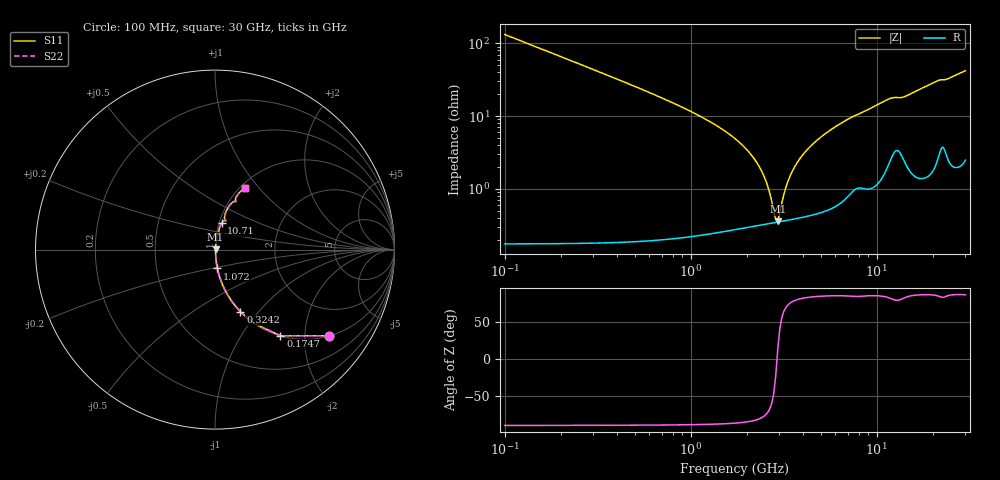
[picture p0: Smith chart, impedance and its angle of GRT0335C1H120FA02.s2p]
!Murata Part Number: GRT0335C1H120FA02
!These Parameters are Measured in Series Mode Connection
!Data Generated on Jun 19, 2026
!  o--ll--o
!Port1  Port2
!  o------o
!Operation Temp=25[degC], DC Bias Voltage=0[V]
!Freq. Start=100[MHz] Stop=30[GHz] 401[Steps]
# Hz S RI R 50
!Freq.(Hz) S11(Real) S11(Imag) S21(Real) S21(Imag) S12(Real) S12(Imag) S22(Real) S22(Imag)
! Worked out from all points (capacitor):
!   401 points, 100 MHz to 30 GHz, reference 50 ohm
!   read as one part in series: C = 12 pF near 249.5 MHz
!   lowest |Z| = 360 mohm at 2.941 GHz (marker M1)
!   series resonance near 2.915 GHz, so ESL is about 250 pH
!   S11 on the Smith chart (normalised r, x): 100 MHz: 1.00, -2.65; 174.8 MHz: 1.00, -1.51; 324.2 MHz: 1.00, -0.81; 1.072 GHz: 1.00, -0.21; 10.71 GHz: 1.03, +0.31; 30 GHz: 1.05, +0.84
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1e8  0.6368 -0.4803  0.3632 0.4803  0.3632 0.4803  0.6368 -0.4803
1.7475e8  0.3641 -0.48  0.6359 0.48  0.6359 0.48  0.3641 -0.48
3.2425e8  0.1413 -0.3461  0.8587 0.3461  0.8587 0.3461  0.1413 -0.3461
5.485e8  0.0531 -0.2201  0.9469 0.2201  0.9469 0.2201  0.0531 -0.2201
1.07175e9  0.0134 -0.1049  0.9866 0.1049  0.9866 0.1049  0.0134 -0.1049
2.193e9  0.00373 -0.0258  0.9963 0.0258  0.9963 0.0258  0.00373 -0.0258
2.492e9  0.00344 -0.0141  0.9966 0.0141  0.9966 0.0141  0.00344 -0.0141
2.791e9  0.00343 -0.00388  0.9966 0.00388  0.9966 0.00388  0.00343 -0.00388
2.9405e9  0.0035 0.000787  0.9965 -0.000787  0.9965 -0.000787  0.0035 0.000787
3.01525e9  0.00355 0.00303  0.9965 -0.00303  0.9965 -0.00303  0.00355 0.00303
3.2395e9  0.00375 0.00945  0.9963 -0.00945  0.9963 -0.00945  0.00375 0.00945
3.389e9  0.00392 0.0135  0.9961 -0.0135  0.9961 -0.0135  0.00392 0.0135
3.688e9  0.00435 0.0212  0.9957 -0.0212  0.9957 -0.0212  0.00435 0.0212
4.286e9  0.00547 0.0352  0.9945 -0.0352  0.9945 -0.0352  0.00547 0.0352
5.10825e9  0.00757 0.0527  0.9924 -0.0527  0.9924 -0.0527  0.00757 0.0527
6.977e9  0.0156 0.0879  0.9844 -0.0879  0.9844 -0.0879  0.0156 0.0879
1.01165e10  0.0311 0.1376  0.9689 -0.1376  0.9689 -0.1376  0.0311 0.1376
1.07145e10  0.0366 0.1472  0.9634 -0.1472  0.9634 -0.1472  0.0366 0.1472
1.505e10  0.0535 0.1849  0.9465 -0.1849  0.9465 -0.1849  0.0535 0.1849
2.005825e10  0.0889 0.2554  0.9111 -0.2554  0.9111 -0.2554  0.0889 0.2554
2.50665e10  0.119 0.2937  0.881 -0.2937  0.881 -0.2937  0.119 0.2937
3e10  0.1649 0.3428  0.8351 -0.3428  0.8351 -0.3428  0.1649 0.3428
